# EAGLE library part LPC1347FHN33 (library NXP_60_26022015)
32-bit ARM Cortex-M3 microcontroller; up to 64 kB flash; up to 12 kB SRAM; USB device; USART; EEPROM The LPC1315/16/17/45/46/47 are ARM Cortex-M3 based microcontrollers for embedded applications featuring a high level of integration and low power consumption. The ARM Cortex-M3 is a next generation core that offers system enhancements such as enhanced debug features and a higher level of support block integration. The LPC1315/16/17/45/46/47 operate at CPU frequencies of up to 72 MHz. The ARM Cortex-M3 CPU incorporates a 3-stage pipeline and uses a Harvard architecture with separate local instruction and data buses as well as a third bus for peripherals. The ARM Cortex-M3 CPU also includes an internal prefetch unit that supports speculative branching. Equipped with a highly flexible and configurable Full-Speed USB 2.0 device controller available on the LPC1345/46/47, this series brings unparalleled design flexibility and seamless integration to today’s demanding connectivity solutions. The peripheral complement of the LPC1315/16/17/45/46/47 includes up to 64 kB of flash memory, 8 kB or 10 kB of SRAM data memory, one Fast-mode Plus I 2 C-bus interface, one RS-485/EIA-485 USART with support for synchronous mode and smart card interface, two SSP interfaces, four general purpose counter/timers, an 8-channel, 12-bit ADC, and up to 51 general purpose I/O pins. AAL Eindhoven MK
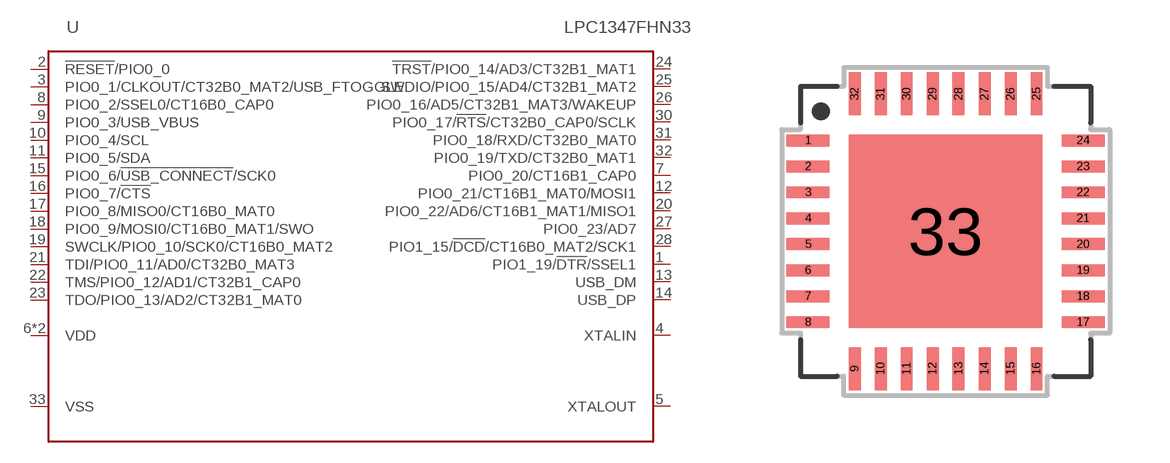
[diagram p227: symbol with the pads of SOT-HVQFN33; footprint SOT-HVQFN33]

Designator prefix U

## LPC1347FHN33 (EEPROM: 4kB; FLASH: 64kB; GPIO: 26; SRAM0: 8kB; SRAM1: 2kB; SRAM_USB: 2kB; USB: yes)  [SOT-HVQFN33]
1  PIO1_19/!DTR!/SSEL1
2  !RESET!/PIO0_0
3  PIO0_1/CLKOUT/CT32B0_MAT2/USB_FTOGGLE
4  XTALIN  in
5  XTALOUT  out
6  VDD  pwr
7  PIO0_20/CT16B1_CAP0
8  PIO0_2/SSEL0/CT16B0_CAP0
9  PIO0_3/USB_VBUS
10  PIO0_4/SCL
11  PIO0_5/SDA
12  PIO0_21/CT16B1_MAT0/MOSI1
13  USB_DM
14  USB_DP
15  PIO0_6/!USB_CONNECT!/SCK0
16  PIO0_7/!CTS!
17  PIO0_8/MISO0/CT16B0_MAT0
18  PIO0_9/MOSI0/CT16B0_MAT1/SWO
19  SWCLK/PIO0_10/SCK0/CT16B0_MAT2
20  PIO0_22/AD6/CT16B1_MAT1/MISO1
21  TDI/PIO0_11/AD0/CT32B0_MAT3
22  TMS/PIO0_12/AD1/CT32B1_CAP0
23  TDO/PIO0_13/AD2/CT32B1_MAT0
24  !TRST!/PIO0_14/AD3/CT32B1_MAT1
25  SWDIO/PIO0_15/AD4/CT32B1_MAT2
26  PIO0_16/AD5/CT32B1_MAT3/WAKEUP
27  PIO0_23/AD7
28  PIO1_15/!DCD!/CT16B0_MAT2/SCK1
29  VDD  pwr
30  PIO0_17/!RTS!/CT32B0_CAP0/SCLK
31  PIO0_18/RXD/CT32B0_MAT0
32  PIO0_19/TXD/CT32B0_MAT1
33  VSS  pwr

## Footprint SOT-HVQFN33 (pad centres in mm)
SOTxxx HVQFN33: plastic thermal enhanced very thin quad flat package; no leads; 33 terminals; body 7 x 7 x 0.85 mm JEDEC: --- IEC: --- Package according LPC111x datasheet
smd 1.075 x 0.3: 1 -3.438,2.275; 2 -3.438,1.625; 3 -3.438,0.975; 4 -3.438,0.325; 5 -3.438,-0.325; 6 -3.438,-0.975; 7 -3.438,-1.625; 8 -3.438,-2.275; 17 3.438,-2.275; 18 3.438,-1.625; 19 3.438,-0.975; 20 3.438,-0.325; 21 3.438,0.325; 22 3.438,0.975; 23 3.438,1.625; 24 3.438,2.275
smd 0.3 x 1.075: 9 -2.275,-3.438; 10 -1.625,-3.438; 11 -0.975,-3.438; 12 -0.325,-3.438; 13 0.325,-3.438; 14 0.975,-3.438; 15 1.625,-3.438; 16 2.275,-3.438; 25 2.275,3.438; 26 1.625,3.438; 27 0.975,3.438; 28 0.325,3.438; 29 -0.325,3.438; 30 -0.975,3.438; 31 -1.625,3.438; 32 -2.275,3.438
smd 4.85 x 4.85: 33 0,0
